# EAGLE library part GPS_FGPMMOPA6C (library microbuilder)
FGPMMOPA6C 16x16 GPS Module NMEA Sentences: GGA, GSA, GSV, RMC, VTG
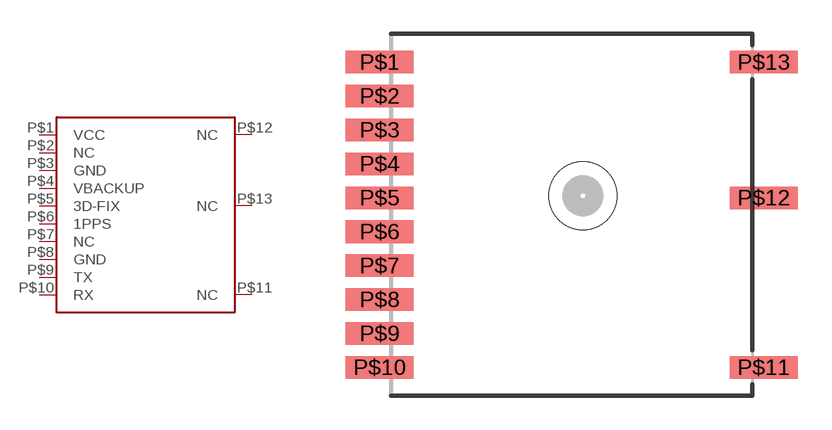
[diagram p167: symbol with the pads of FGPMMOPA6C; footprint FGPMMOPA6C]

Designator prefix U

## GPS_FGPMMOPA6C  [FGPMMOPA6C]
P$1  VCC
P$2  NC
P$3  GND
P$4  VBACKUP
P$5  3D-FIX
P$6  1PPS
P$7  NC
P$8  GND
P$9  TX
P$10  RX
P$11  NC
P$12  NC
P$13  NC

## Footprint FGPMMOPA6C (pad centres in mm)
smd 3 x 1: P$1 -8.5,6.75; P$2 -8.5,5.25; P$3 -8.5,3.75; P$4 -8.5,2.25; P$5 -8.5,0.75; P$6 -8.5,-0.75; P$7 -8.5,-2.25; P$8 -8.5,-3.75; P$9 -8.5,-5.25; P$10 -8.5,-6.75; P$11 8.5,-6.75; P$12 8.5,0.75; P$13 8.5,6.75
hole 3 at 0.5,0.85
